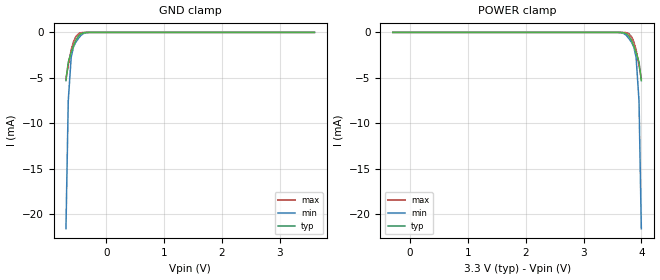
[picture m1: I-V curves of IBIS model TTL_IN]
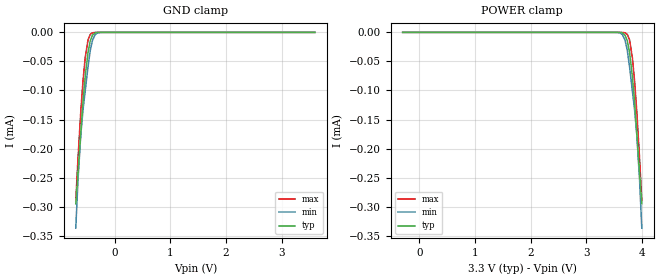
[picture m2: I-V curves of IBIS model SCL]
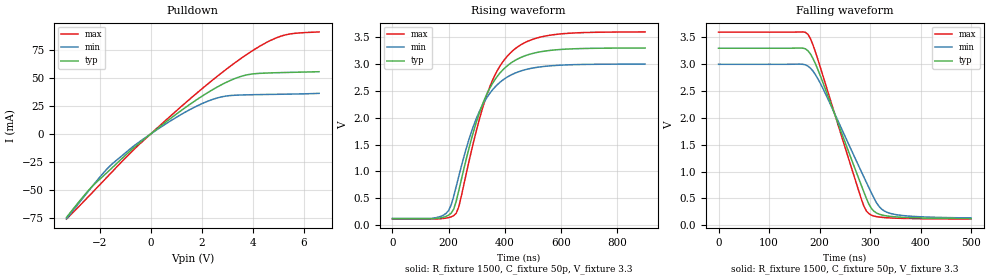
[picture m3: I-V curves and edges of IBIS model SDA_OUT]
[IBIS Ver]   3.2
[Comment Char]   |_char
[File name]   pca9530_3_3v.ibs
[File Rev]   1
[Date]   Nov 19, 2008 3:45:29 PM
[Source]
Generated by Seshadri Venkataramanan using IBIS Toolkit at NXP Tempe
[Notes]
[Disclaimer]
(C) Copyright 2007 NXP Semiconductors
All rights reserved
NXP Semiconductors (NXP) does not warrant that this model and any other
accompanying information (Model) accurately or fully represents the
operating characteristics and specifications of the semiconductor
products to which the Model relates.  Moreover, the Model is furnished
on an "as is" and with "all faults" basis, and without support or
warranty of any kind.  NXP disclaims all warranties, whether expressed
or implied or statutory, including without limitation all implied
warranties of non-infringement, merchantability and fitness for any
purpose, and those arising from a course of dealing or usage of trade.
NXP does not convey any license under its or any third party's patents,
copyrights or other intellectual property or proprietary rights.
You and your company assume any and all risks and liability arising out
of the application or use of the Model.
In no event shall NXP be liable for any direct, indirect, special,
consequential or incidental damages, however caused, whether in
warranty, contract or tort (including negligence), strict liability or
other legal theory, including, without limitation, for lost profits,
business interruption, or corruption or loss of data or information,
arising out of or in connection with the use of or the inability to use
the Model, even if NXP has been advised of the possibility of such
damages.
NXP provides the Model as a courtesy to our customers. You and your
company shall not distribute, convey, sell, or give the Model to anyone
else without receiving prior written permission from NXP.
NXP reserves the right to make changes without notice to the Model to
improve reliability, function, or design.
Please be aware that your receipt and subsequent use of the Model shall
serve as acceptance of these terms and conditions.  If you do not
accept these terms, return or destroy the Model immediately.
[Copyright]
2008
[Component]   PCA9530D
Si_location Pin
Timing_location Pin
[Manufacturer]   NXP Semiconductors
[Package]
R_pkg   4.81E-02   4.14E-02   5.47E-02
L_pkg   1.88E-09   1.54E-09   2.21E-09
C_pkg   4.49E-13   4.17E-13   4.81E-13
[Pin] signal_name   model_name   R_pin   L_pin   C_pin
1   A0   TTL_IN   5.47E-02  2.21E-09  4.81E-13
2   LED0   LED_OUT   4.14E-02  1.54E-09  4.20E-13
3   LED1   LED_OUT   4.14E-02  1.55E-09  4.20E-13
4   Vss   GND   5.47E-02  2.21E-09  4.80E-13
5   RESETb   TTL_IN   5.47E-02  2.21E-09  4.78E-13
6   SCL   SCL   4.14E-02  1.55E-09  4.17E-13
7   SDA   SDA   4.14E-02  1.54E-09  4.17E-13
8   VDD   POWER   5.47E-02  2.21E-09  4.79E-13
[Component]   PCA9530DP
Si_location Pin
Timing_location Pin
[Manufacturer]   NXP Semiconductors
[Package]
R_pkg   33.7m   30.1m   37.3m
L_pkg   1.74n   1.67n   1.81n
C_pkg   0.428p   0.422p   0.434p
[Pin] signal_name   model_name   R_pin   L_pin   C_pin
1   A0   TTL_IN   37.3m   1.81nH   0.428pF
2   LED0   LED_OUT   30.1m   1.67nH   0.422pF
3   LED1   LED_OUT   30.1m   1.67nH   0.428pF
4   Vss   GND   37.3m   1.81nH   0.434pF
5   RESETb   TTL_IN   37.3m   1.81nH   0.428pF
6   SCL   SCL   30.1m   1.67nH   0.422pF
7   SDA   SDA   30.1m   1.67nH   0.428pF
8   VDD   POWER   37.3m   1.81nH   0.434pF
[Model Selector]   SDA
SDA_IN   SDA Input
SDA_OUT   SDA output
| Models and submodels in the file (5): TTL_IN (Input), SCL (Input), SDA_OUT (Open_drain), LED_OUT (Open_drain), SDA_IN (Input)
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[Model]   TTL_IN
Model_type Input
Vinh=2.31
Vinl=0.99
C_comp   1.73p   1.7p   1.75p
[Temperature Range] 27   85   -40
[Voltage Range]   3.3   3   3.6
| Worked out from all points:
|   GND clamp passes 1 mA (typ) near -0.54 V on its own axis
[GND Clamp]
-700mV    -5.302mA   -21.58mA   -5.122mA
-660mV    -3.272mA   -7.517mA   -3.572mA
-610mV    -2.203mA   -2.754mA   -1.946mA
-570mV    -1.517mA   -1.6mA     -1.043mA
-530mV    -870.3uA   -1.076mA   -474.7uA
-480mV    -358.1uA   -640.7uA   -129.8uA
-440mV    -144.9uA   -321.1uA   -35.11uA
-350mV    -9.525uA   -35.75uA   -921.4nA
-270mV    -463.2nA   -2.623uA   -22.77nA
3.6V      65.11pA    250.9pA    47.06pA
[POWER Clamp]
-300mV    65.11pA    250.9pA    47.06pA
3.57V     -463.2nA   -2.623uA   -22.77nA
3.65V     -9.525uA   -35.75uA   -921.4nA
3.74V     -144.9uA   -321.1uA   -35.11uA
3.78V     -358.1uA   -640.7uA   -129.8uA
3.83V     -870.3uA   -1.076mA   -474.7uA
3.87V     -1.517mA   -1.6mA     -1.043mA
3.91V     -2.203mA   -2.754mA   -1.946mA
3.96V     -3.272mA   -7.517mA   -3.572mA
4V        -5.302mA   -21.58mA   -5.122mA
[Model]   SCL
Model_type Input
Vinh=2.31
Vinl=0.99
C_comp   3p   2.8p   3.2p
[Temperature Range] 27   85   -40
[Voltage Range]   3.3   3   3.6
[GND Clamp]
-700mV    -295uA     -337uA     -289.5uA
-660mV    -241.9uA   -254.1uA   -216.6uA
-610mV    -172.6uA   -176.5uA   -136.3uA
-570mV    -119.6uA   -133.4uA   -83.31uA
-530mV    -75.1uA    -100.5uA   -43.1uA
-480mV    -34.54uA   -59.09uA   -13.06uA
-440mV    -14.75uA   -31.48uA   -3.492uA
-400mV    -4.926uA   -13.83uA   -710.6nA
-350mV    -920.5nA   -3.647uA   -77.68nA
-310mV    -204.4nA   -1.016uA   -12.1nA
-220mV    -5.506nA   -39.51nA   -164pA
3.6V      8.544pA    24.57pA    7.213pA
[POWER Clamp]
-300mV    8.544pA    24.57pA    7.213pA
3.52V     -5.506nA   -39.51nA   -164pA
3.61V     -204.4nA   -1.016uA   -12.1nA
3.65V     -920.5nA   -3.647uA   -77.68nA
3.7V      -4.926uA   -13.83uA   -710.6nA
3.74V     -14.75uA   -31.48uA   -3.492uA
3.78V     -34.54uA   -59.09uA   -13.06uA
3.83V     -75.1uA    -100.5uA   -43.1uA
3.87V     -119.6uA   -133.4uA   -83.31uA
3.91V     -172.6uA   -176.5uA   -136.3uA
3.96V     -241.9uA   -254.1uA   -216.6uA
4V        -295uA     -337uA     -289.5uA
[Model]   SDA_OUT
Model_type Open_drain
Vref=3.3
Vmeas=1.65
Rref=1.5k
Cref=50p
C_comp   4p   3.8p   4.2p
[Temperature Range] 27   85   -40
[Voltage Range]   3.3   3   3.6
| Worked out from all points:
|   slope of the pulldown table from 0 to 0.495 V, typ, clamps not added: 55.4 ohm
|   falling waveform, R_fixture 1500, C_fixture 50p, V_fixture 3.3: 20-80 % time 75.6ns typ, 84.3ns min, 68.9ns max; typ from 3.3 V to 0.123 V
|   rising waveform, R_fixture 1500, C_fixture 50p, V_fixture 3.3: 20-80 % time 118ns typ, 117ns min, 119ns max; typ from 0.116 V to 3.3 V
[Pulldown]
-3.3V     -74.78mA   -76.07mA   -76.19mA
-2.4V     -49.61mA   -50.07mA   -55.18mA
-1.5V     -30.06mA   -26.65mA   -33.63mA
-600mV    -11.14mA   -9.676mA   -12.65mA
100mV     1.828mA    1.566mA    2.093mA
1.8V      30.66mA    24.91mA    36.45mA
2.6V      41.96mA    32.21mA    51.49mA
3.3V      49.67mA    34.73mA    63.75mA
3.9V      53.51mA    35.15mA    73.3mA
4.6V      54.66mA    35.44mA    82.73mA
5.4V      55.18mA    35.72mA    89.38mA
6.6V      55.81mA    36.43mA    91.45mA
[Falling Waveform]
R_fixture=1500
C_fixture=50p
V_fixture=3.3
V_fixture_min=3
V_fixture_max=3.6
0s        3.3V       3V         3.6V
161.6ns   3.303V     3.003V     3.603V
176.8ns   3.256V     2.968V     3.562V
186.9ns   3.111V     2.875V     3.365V
202ns     2.774V     2.637V     2.929V
282.8ns   739.3mV    996.7mV    484.7mV
298ns     385.8mV    693.9mV    211.9mV
318.2ns   204.5mV    345.4mV    151.6mV
338.4ns   166.2mV    224.2mV    135.7mV
500ns     123.2mV    135.1mV    114.8mV
[Rising Waveform]
R_fixture=1500
C_fixture=50p
V_fixture=3.3
V_fixture_min=3
V_fixture_max=3.6
0s        116.1mV    122.6mV    111.1mV
181.8ns   144.6mV    183.7mV    121.9mV
209.1ns   220.5mV    373.1mV    151.4mV
227.3ns   447.6mV    721.9mV    221mV
281.8ns   1.614V     1.745V     1.395V
327.3ns   2.335V     2.298V     2.287V
381.8ns   2.826V     2.655V     2.953V
445.5ns   3.094V     2.85V      3.319V
581.8ns   3.265V     2.975V     3.553V
900ns     3.299V     2.999V     3.599V
[Ramp]
R_load=1500
dV/dt_r   1.910E+0/7.439E-8   1.899E+0/7.271E-8   1.919E+0/7.565E-8
dV/dt_f   1.906E+0/7.492E-8   1.891E+0/9.127E-8   1.917E+0/6.297E-8
|[End   SDA_OUT
